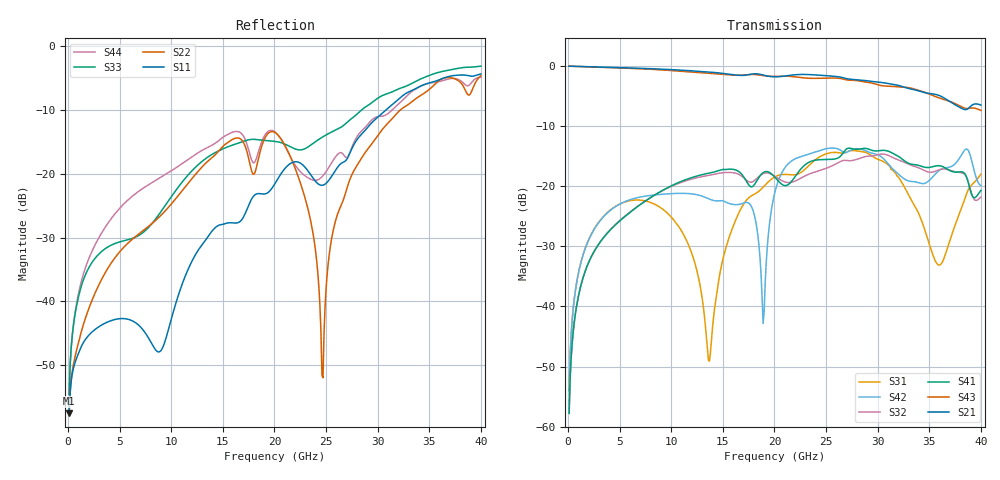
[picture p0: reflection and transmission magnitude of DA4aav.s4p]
! ADC12DJ2700AAV, ADC12DJ3200AAV, ADC08DJ3200AAV
! 144 pin AAV package
! Texas Instruments 4/21/2021
! Single-ended  S-parameters
! PORT#  PORT_NAME  NET_NAME
! PORT1:  DAxN.DIEBUMP DAxN
! PORT2:  DAxN.BGA  DAxN
! PORT3:  DAxP.DIEBUMP DAxP
! PORT4:  DAxP.BGA  DAxP
! Touchstone Ver. 1.0
! Number of ports is 4
# Hz	S	MA	R	50.000000
! SCATTERING PARAMETERS  :
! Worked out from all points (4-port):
!   400 points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, 100 MHz to 40 GHz, reference 50 ohm
!   strongest paths, dB at 100 MHz, 10.1 GHz, 20.1 GHz, 30.1 GHz, 40 GHz:
!     S21: 0.0, -0.6, -1.8, -2.7, -6.5
!     S43: 0.0, -0.8, -1.7, -3.1, -7.4
!     S41: -57.8, -19.8, -18.6, -14.1, -20.7
!     S32: -57.8, -19.9, -18.4, -14.7, -21.8
!     S42: -54.0, -21.2, -20.6, -14.8, -19.9
!     S31: -54.0, -25.3, -18.4, -15.6, -18.0
!   lowest |S11| = -57.6 dB at 100 MHz (marker M1), VSWR 1.00, Z = 50.1 + j0.0719 ohm
!   |S11| at or under -10 dB: start of sweep to 30.77 GHz
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1e8  0.001319 33.0  0.9986 -1.0  0.001993 85.6  0.00129 -95.9
     0.9986 -1.0  0.001326 32.2  0.00129 -95.9  0.001992 85.5
     0.001993 85.6  0.00129 -95.9  0.001864 56.0  0.9987 -1.0
     0.00129 -95.9  0.001992 85.5  0.9987 -1.0  0.001873 55.0
4e9  0.00696 -21.8  0.9765 -38.6  0.06253 42.9  0.04247 -140.9
     0.9765 -38.6  0.01895 -37.3  0.0428 -140.6  0.06204 44.4
     0.06253 42.9  0.0428 -140.6  0.02708 53.1  0.9718 -37.2
     0.04247 -140.9  0.06204 44.4  0.9718 -37.2  0.0425 -2.1
1.37e10  0.03341 10.6  0.8905 -130.2  0.003504 -149.2  0.1288 110.0
         0.8905 -130.2  0.1289 -68.3  0.1234 110.4  0.07818 -41.5
         0.003504 -149.2  0.1234 110.4  0.1381 55.3  0.8708 -124.0
         0.1288 110.0  0.07818 -41.5  0.8708 -124.0  0.1637 -86.7
1.83e10  0.06967 -10.0  0.8623 -171.5  0.08845 91.6  0.1116 67.9
         0.8623 -171.5  0.1169 -95.2  0.1166 66.6  0.04445 61.0
         0.08845 91.6  0.1166 66.6  0.1856 18.4  0.8476 -163.8
         0.1116 67.9  0.04445 61.0  0.8476 -163.8  0.1362 -119.9
2.47e10  0.08147 -40.4  0.8363 126.8  0.1816 50.5  0.1668 8.0
         0.8363 126.8  0.002507 -60.2  0.1381 15.0  0.2022 30.3
         0.1816 50.5  0.1381 15.0  0.1954 13.5  0.793 139.4
         0.1668 8.0  0.2022 30.3  0.793 139.4  0.09667 66.9
2.76e10  0.1638 -21.1  0.7741 96.6  0.1984 20.8  0.2048 -28.0
         0.7741 96.6  0.1022 -25.0  0.1643 -17.4  0.2025 -9.5
         0.1984 20.8  0.1643 -17.4  0.2765 9.8  0.7626 110.1
         0.2048 -28.0  0.2025 -9.5  0.7626 110.1  0.1693 -7.8
4e10  0.6086 -141.8  0.4739 -25.8  0.1261 127.3  0.09231 -155.8
      0.4739 -25.8  0.5885 -96.9  0.08134 -142.3  0.1012 86.1
      0.1261 127.3  0.08134 -142.3  0.6997 -93.1  0.4277 -7.9
      0.09231 -155.8  0.1012 86.1  0.4277 -7.9  0.5711 -112.5
